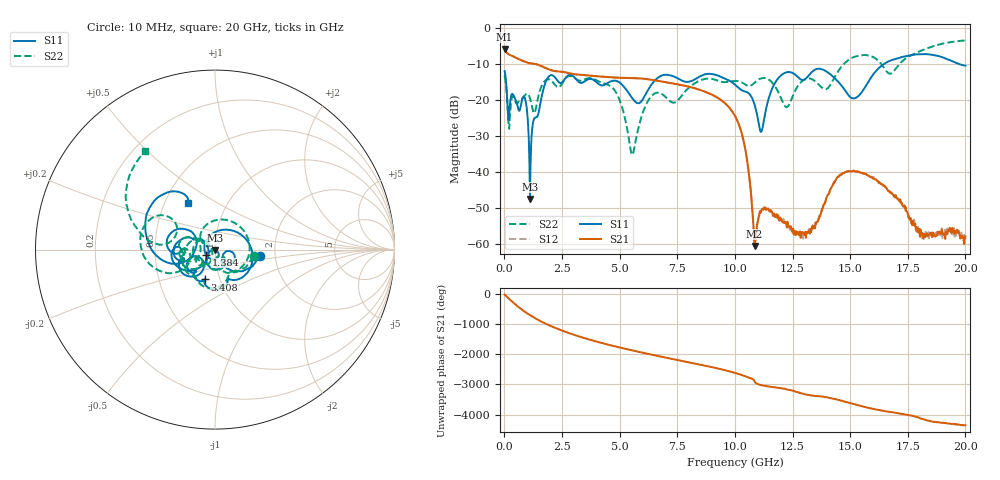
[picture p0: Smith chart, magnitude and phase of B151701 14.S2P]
!  2-Port S-parameters saved by WinCal
! VAR MeasName=S-Parameters (CALIBRATED_DATA) read from VNA (N5244A)
! VAR MeasDate=2015-12-24 19:09:44
! VAR NAME=B151701 14
! VAR FILENAME=B151701 14.S2P
! VAR DATE=2015-12-24 19:09:44
! VAR PHYS_PORTS=1,3
# Hz S DB R 50
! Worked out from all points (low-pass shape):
!   801 points, 10 MHz to 20 GHz, reference 50 ohm
!   highest |S21| = -5.80 dB at 10 MHz (marker M1); lowest = -60.5 dB at 10.85 GHz (marker M2)
!   |S21| within 3 dB of the highest: start of sweep to 677.1 MHz
!   lowest |S11| = -47.4 dB at 1.109 GHz (marker M3), VSWR 1.01, Z = 49.9 - j0.402 ohm
!   |S11| at or under -10 dB: start of sweep to 16.47 GHz; 19.72 GHz to end of sweep
!   |S22| runs from -35.2 to -3.5 dB; largest |S21 - S12| = 0.0017
!   S11 on the Smith chart (normalised r, x): 10 MHz: 1.66, -0.12; 1.384 GHz: 0.90, -0.05; 3.408 GHz: 0.85, -0.29; 20 GHz: 0.65, +0.37
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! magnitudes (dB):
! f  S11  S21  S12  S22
! 10 MHz  -11.9  -5.8  -5.8  -13.2
! 209.9 MHz  -23.9  -7.4  -7.4  -28.0
! 884.6 MHz  -19.4  -9.3  -9.3  -18.7
! 1.109 GHz  -47.4  -9.8  -9.8  -19.5
! 1.384 GHz  -24.8  -10.1  -10.1  -21.7
! 1.959 GHz  -13.3  -11.6  -11.6  -14.3
! 3.358 GHz  -15.2  -13.0  -13.0  -14.6
! 3.408 GHz  -15.1  -13.0  -13.0  -14.5
! 4.783 GHz  -14.6  -13.8  -13.8  -17.3
! 5.557 GHz  -19.6  -13.9  -13.9  -35.2
! 6.682 GHz  -13.7  -14.7  -14.7  -17.9
! 10.01 GHz  -15.7  -24.4  -24.4  -14.7
! 10.48 GHz  -17.7  -34.7  -34.6  -15.8
! 10.85 GHz  -21.2  -60.5  -60.5  -15.2
! 11.15 GHz  -28.6  -50.5  -50.5  -13.9
! 11.93 GHz  -13.6  -53.4  -53.0  -18.4
! 13.35 GHz  -12.1  -55.1  -55.6  -14.2
! 14.7 GHz  -16.6  -40.2  -40.4  -10.1
! 15.28 GHz  -19.3  -39.9  -39.8  -7.8
! 16.68 GHz  -9.2  -45.1  -45.1  -12.6
! 18.15 GHz  -7.3  -57.4  -56.9  -6.1
! 20 GHz  -10.5  -57.8  -58.7  -3.5
